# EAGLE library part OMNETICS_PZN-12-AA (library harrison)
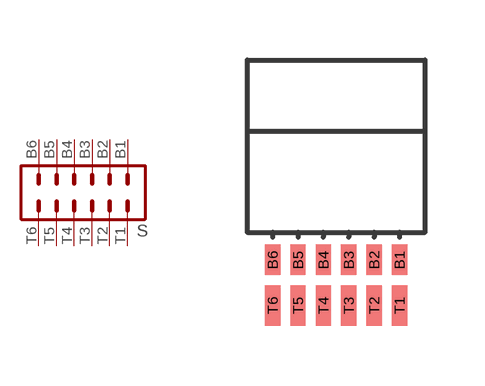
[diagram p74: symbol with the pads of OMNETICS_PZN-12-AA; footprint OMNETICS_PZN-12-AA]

Designator prefix S

## OMNETICS_PZN-12-AA  [OMNETICS_PZN-12-AA]
B1  B1  pas
B2  B2  pas
B3  B3  pas
B4  B4  pas
B5  B5  pas
B6  B6  pas
T1  T1  pas
T2  T2  pas
T3  T3  pas
T4  T4  pas
T5  T5  pas
T6  T6  pas

## Footprint OMNETICS_PZN-12-AA (pad centres in mm)
smd 0.381 x 0.762: B1 1.587,-1.016; B2 0.953,-1.016; B3 0.318,-1.016; B4 -0.318,-1.016; B5 -0.953,-1.016; B6 -1.587,-1.016
smd 0.381 x 1.016: T1 1.587,-2.159; T2 0.953,-2.159; T3 0.318,-2.159; T4 -0.318,-2.159; T5 -0.953,-2.159; T6 -1.587,-2.159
